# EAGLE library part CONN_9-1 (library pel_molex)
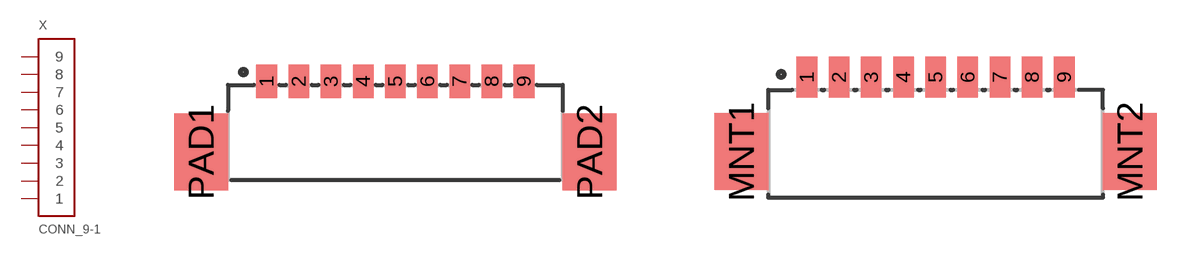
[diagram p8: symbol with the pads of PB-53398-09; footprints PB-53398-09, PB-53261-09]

Designator prefix X

## CONN_9-1-53398  [PB-53398-09]
1  1
2  2
3  3
4  4
5  5
6  6
7  7
8  8
9  9

## CONN_9-1-53261  [PB-53261-09]
Pads as for PB-53398-09

## CONN_9-1-53047  [PB-53047-09]
Pads as for PB-53398-09

## Footprint PB-53398-09 (pad centres in mm)
smd 0.8 x 1.3: 1 -5,1.25; 2 -3.75,1.25; 3 -2.5,1.25; 4 -1.25,1.25; 5 0,1.25; 6 1.25,1.25; 7 2.5,1.25; 8 3.75,1.25; 9 5,1.25
smd 2.1 x 3: PAD1 -7.55,-1.5; PAD2 7.55,-1.5

## Footprint PB-53261-09 (pad centres in mm)
smd 0.8 x 1.6: 1 -5,1.1; 2 -3.75,1.1; 3 -2.5,1.1; 4 -1.25,1.1; 5 0,1.1; 6 1.25,1.1; 7 2.5,1.1; 8 3.75,1.1; 9 5,1.1
smd 2.1 x 3: MNT1 -7.55,-1.8; MNT2 7.55,-1.8

## Footprint PB-53047-09 (pad centres in mm)
drill 0.5: 1 -5,0; 2 -3.75,0; 3 -2.5,0; 4 -1.25,0; 5 0,0; 6 1.25,0; 7 2.5,0; 8 3.75,0; 9 5,0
